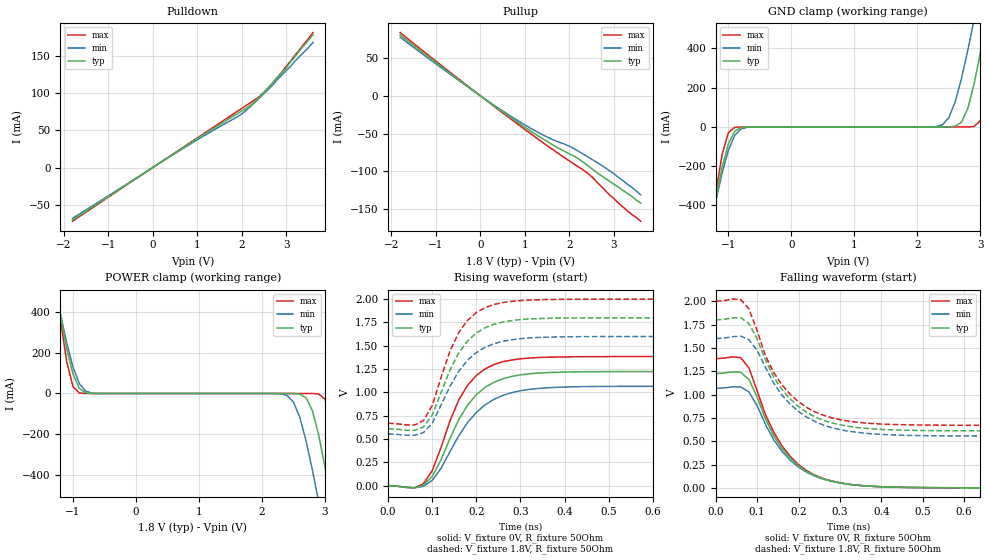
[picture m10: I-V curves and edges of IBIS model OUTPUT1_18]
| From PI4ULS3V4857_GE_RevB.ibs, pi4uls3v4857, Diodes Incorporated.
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[Model]  OUTPUT1_18
Model_type  Output
Vmeas=0.9
|Variable   typ   min   max
C_comp   3.79p   3.76p   3.83p
|Variable   typ   min   max
[Voltage Range]   1.8   1.6   2.0
[Temperature Range]   40   85   -40
[Pullup Reference]   1.8   1.6   2.0
[Pulldown Reference]   0   0   0
[Power Clamp Reference]   1.8   1.6   2.0
[GND Clamp Reference]   0   0   0
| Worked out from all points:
|   slope of the pulldown table from 0 to 0.27 V, typ, clamps not added: 25.4 ohm
|   slope of the pullup table from 0 to 0.27 V, typ, clamps not added: 23.2 ohm
|   GND clamp passes 1 mA (typ) near -0.72 V on its own axis
|   POWER clamp passes 1 mA (typ) near -0.72 V on its own axis
|   falling waveform, V_fixture 0V, R_fixture 50Ohm: 20-80 % time 98.6ps typ, 100ps min, 99.2ps max; typ from 1.22 V to 0 V
|   falling waveform, V_fixture 1.8V, R_fixture 50Ohm: 20-80 % time 104ps typ, 109ps min, 101ps max; typ from 1.8 V to 0.61 V
|   rising waveform, V_fixture 0V, R_fixture 50Ohm: 20-80 % time 84.6ps typ, 93.3ps min, 76.7ps max; typ from 0 V to 1.22 V
|   rising waveform, V_fixture 1.8V, R_fixture 50Ohm: 20-80 % time 75ps typ, 81.6ps min, 69.1ps max; typ from 0.61 V to 1.8 V
[GND Clamp]
-1.8V     -1.56A     -1.42A     -1.93A
-1.3V     -542mA     -535mA     -571mA
-1.1V     -205mA     -235mA     -140mA
-1V       -84.8mA    -118mA     -28.6mA
-900mV    -21.7mA    -42.8mA    -2.29mA
2.4V      6.93uA     11.7mA     8.52pA
2.7V      24.8mA     248mA      315nA
2.9V      220mA      548mA      2.33mA
3V        380mA      713mA      33mA
3.1V      561mA      885mA      156mA
3.3V      951mA      1.24A      608mA
3.6V      1.57A      1.79A      1.43A
[POWER Clamp]
-1.8V     1.57A      1.42A      2.01A
-1.3V     561mA      548mA      608mA
-1V       94.6mA     129mA      33mA
-900mV    24.8mA     48.5mA     2.33mA
-700mV    214uA      1.65mA     315nA
2.4V      -9.58uA    -10.4mA    -8.58pA
2.7V      -21.7mA    -235mA     -455nA
2.9V      -205mA     -535mA     -2.29mA
3V        -363mA     -702mA     -28.6mA
3.1V      -542mA     -876mA     -140mA
3.3V      -932mA     -1.24A     -571mA
3.6V      -1.56A     -1.8A      -1.37A
[Pulldown]
| Voltage   I(typ)   I(min)  I(max)
-1.8V     -70.3mA    -68.1mA    -72mA
700mV     27.3mA     26.3mA     27.8mA
1.9V      72.3mA     68mA       75.4mA
2V        75.9mA     71.9mA     79.3mA
2.2V      83.6mA     82.2mA     87.2mA
2.4V      94.7mA     93.5mA     95.3mA
2.6V      107mA      105mA      107mA
3V        134mA      130mA      136mA
3.3V      157mA      149mA      158mA
3.6V      178mA      168mA      181mA
[Pullup]   |Note: Vtable = Vcc - Voutput
| Voltage   I(typ)   I(min)  I(max)
-1.8V     80.4mA     77.4mA     83.6mA
-600mV    26.3mA     25.1mA     27.4mA
600mV     -25.5mA    -23.9mA    -27mA
1.3V      -53.2mA    -48.5mA    -57.5mA
1.6V      -64mA      -57.3mA    -70.1mA
2V        -76.9mA    -66.8mA    -86.3mA
2.2V      -83.2mA    -73.3mA    -94mA
2.4V      -91.9mA    -80.3mA    -102mA
3V        -117mA     -103mA     -136mA
3.1V      -121mA     -108mA     -142mA
3.4V      -133mA     -121mA     -157mA
3.6V      -142mA     -131mA     -166mA
[Falling Waveform]
V_fixture = 0V
V_fixture_min = 0V
V_fixture_max = 0V
R_fixture = 50Ohm
C_fixture = 0F
|   Time   V(typ)   V(min)   V(max)
0s        1.224V     1.066V     1.384V
60ps      1.238V     1.081V     1.395V
80ps      1.162V     1.028V     1.286V
120ps     738.3mV    678.7mV    784.9mV
140ps     559.6mV    515.3mV    597.1mV
200ps     235.7mV    222mV      249mV
260ps     95.57mV    92.95mV    99.12mV
320ps     38.65mV    38.73mV    39.68mV
520ps     2.054mV    2.233mV    2.017mV
1.98ns    0V         0V         0V
[Falling Waveform]
V_fixture = 1.8V
V_fixture_min = 1.6V
V_fixture_max = 2.0V
R_fixture = 50Ohm
C_fixture = 0F
|   Time   V(typ)   V(min)   V(max)
0s        1.8V       1.6V       2V
60ps      1.824V     1.626V     2.018V
80ps      1.76V      1.588V     1.918V
120ps     1.37V      1.292V     1.415V
140ps     1.186V     1.122V     1.235V
180ps     951.5mV    894.8mV    1.001V
240ps     760.3mV    709.7mV    813.4mV
320ps     659.9mV    607.5mV    715.1mV
560ps     612.1mV    557mV      670.8mV
1.98ns    610.3mV    554.8mV    669.2mV
[Rising Waveform]
V_fixture = 0V
V_fixture_min = 0V
V_fixture_max = 0V
R_fixture = 50Ohm
C_fixture = 0F
|   Time   V(typ)   V(min)   V(max)
0s        0V         0V         0V
80ps      4.174mV    -7.476mV   20.76mV
100ps     100.3mV    57.04mV    161.4mV
120ps     278.7mV    186.7mV    410.1mV
160ps     706.9mV    534.4mV    917.2mV
180ps     862.9mV    677mV      1.075V
220ps     1.055V     867.6mV    1.252V
280ps     1.171V     997.4mV    1.347V
480ps     1.222V     1.064V     1.383V
1.98ns    1.224V     1.066V     1.384V
[Rising Waveform]
V_fixture = 1.8V
V_fixture_min = 1.6V
V_fixture_max = 2.0V
R_fixture = 50Ohm
C_fixture = 0F
|   Time   V(typ)   V(min)   V(max)
0s        610.3mV    554.8mV    669.2mV
60ps      593.5mV    540mV      649.9mV
80ps      629.5mV    568.3mV    697mV
100ps     756.2mV    669.1mV    859.3mV
140ps     1.238V     1.064V     1.441V
160ps     1.423V     1.226V     1.641V
200ps     1.637V     1.427V     1.856V
260ps     1.755V     1.548V     1.963V
440ps     1.798V     1.598V     1.999V
1.98ns    1.8V       1.6V       2V
[Ramp]
|   typ   min   max
dV/dt_r   0.99/0.96E-10   0.86/0.98E-10   1.12/0.96E-10
dV/dt_f   0.99/0.58E-10   0.87/0.64E-10   1.12/0.52E-10
R_load =   50.0000
